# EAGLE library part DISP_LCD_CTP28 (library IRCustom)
2.83" 240x320 Pixel Capacitive Touch Display
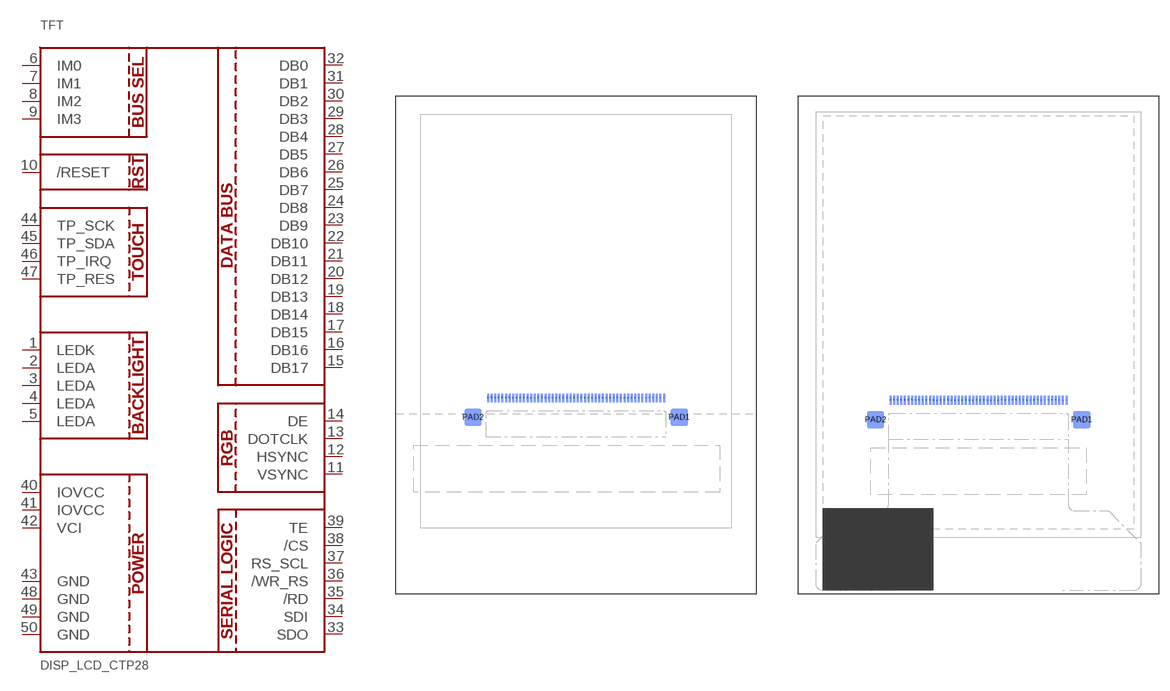
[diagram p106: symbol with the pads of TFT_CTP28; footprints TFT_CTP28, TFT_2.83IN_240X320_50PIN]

Designator prefix TFT

## DISP_LCD_CTP28_DATASHEET  [TFT_CTP28]
1  LEDK
2  LEDA
3  LEDA
4  LEDA
5  LEDA
6  IM0
7  IM1
8  IM2
9  IM3
10  /RESET
11  VSYNC
12  HSYNC
13  DOTCLK
14  DE
15  DB17
16  DB16
17  DB15
18  DB14
19  DB13
20  DB12
21  DB11
22  DB10
23  DB9
24  DB8
25  DB7
26  DB6
27  DB5
28  DB4
29  DB3
30  DB2
31  DB1
32  DB0
33  SDO
34  SDI
35  /RD
36  /WR_RS
37  RS_SCL
38  /CS
39  TE
40  IOVCC
41  IOVCC
42  VCI
43  GND
44  TP_SCK
45  TP_SDA
46  TP_IRQ
47  TP_RES
48  GND
49  GND
50  GND

## DISP_LCD_CTP28_SAMPLE  [TFT_2.83IN_240X320_50PIN]
Pads as for TFT_CTP28

## Footprint TFT_CTP28 (pad centres in mm)
smd 0.275 x 1.2 bottom: 1 12.25,-7.36; 2 11.75,-7.36; 3 11.25,-7.36; 4 10.75,-7.36; 5 10.25,-7.36; 6 9.75,-7.36; 7 9.25,-7.36; 8 8.75,-7.36; 9 8.25,-7.36; 10 7.75,-7.36; 11 7.25,-7.36; 12 6.75,-7.36; 13 6.25,-7.36; 14 5.75,-7.36; 15 5.25,-7.36; 16 4.75,-7.36; 17 4.25,-7.36; 18 3.75,-7.36; 19 3.25,-7.36; 20 2.75,-7.36; 21 2.25,-7.36; 22 1.75,-7.36; 23 1.25,-7.36; 24 0.75,-7.36; 25 0.25,-7.36; 26 -0.25,-7.36; 27 -0.75,-7.36; 28 -1.25,-7.36; 29 -1.75,-7.36; 30 -2.25,-7.36; 31 -2.75,-7.36; 32 -3.25,-7.36; 33 -3.75,-7.36; 34 -4.25,-7.36; 35 -4.75,-7.36; 36 -5.25,-7.36; 37 -5.75,-7.36; 38 -6.25,-7.36; 39 -6.75,-7.36; 40 -7.25,-7.36; 41 -7.75,-7.36; 42 -8.25,-7.36; 43 -8.75,-7.36; 44 -9.25,-7.36; 45 -9.75,-7.36; 46 -10.25,-7.36; 47 -10.75,-7.36; 48 -11.25,-7.36; 49 -11.75,-7.36; 50 -12.25,-7.36
smd 2.4 x 2.4 bottom: PAD1 14.35,-10.06; PAD2 -14.35,-10.06

## Footprint TFT_2.83IN_240X320_50PIN (pad centres in mm)
smd 0.275 x 1.2 bottom: 1 12.25,-10.39; 2 11.75,-10.39; 3 11.25,-10.39; 4 10.75,-10.39; 5 10.25,-10.39; 6 9.75,-10.39; 7 9.25,-10.39; 8 8.75,-10.39; 9 8.25,-10.39; 10 7.75,-10.39; 11 7.25,-10.39; 12 6.75,-10.39; 13 6.25,-10.39; 14 5.75,-10.39; 15 5.25,-10.39; 16 4.75,-10.39; 17 4.25,-10.39; 18 3.75,-10.39; 19 3.25,-10.39; 20 2.75,-10.39; 21 2.25,-10.39; 22 1.75,-10.39; 23 1.25,-10.39; 24 0.75,-10.39; 25 0.25,-10.39; 26 -0.25,-10.39; 27 -0.75,-10.39; 28 -1.25,-10.39; 29 -1.75,-10.39; 30 -2.25,-10.39; 31 -2.75,-10.39; 32 -3.25,-10.39; 33 -3.75,-10.39; 34 -4.25,-10.39; 35 -4.75,-10.39; 36 -5.25,-10.39; 37 -5.75,-10.39; 38 -6.25,-10.39; 39 -6.75,-10.39; 40 -7.25,-10.39; 41 -7.75,-10.39; 42 -8.25,-10.39; 43 -8.75,-10.39; 44 -9.25,-10.39; 45 -9.75,-10.39; 46 -10.25,-10.39; 47 -10.75,-10.39; 48 -11.25,-10.39; 49 -11.75,-10.39; 50 -12.25,-10.39
smd 2.4 x 2.4 bottom: PAD1 14.35,-13.09; PAD2 -14.35,-13.09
